(* Logix 5000 Routine export Bead_Edit_Support; software revision 36.00 *)

TYPE DUT_NDSN_spLink :   // UDDT that holds the Cyclic and ACyclic data for the SpectraLink.
STRUCT
   b_r_LostComm : BOOL;
   b_r_PLC_CommReadOnly : BOOL;
   b_r_SystemReady : BOOL;   // Pattern Status Word 0 Bit 0
   b_r_Fault : BOOL;   // Pattern Status Word 0 Bit 1
   b_r_Alert : BOOL;   // Pattern Status Word 0 Bit 2
   b_r_Commissioned : BOOL;   // Pattern Status Word 0 Bit 3
   b_r_RecipeModified : BOOL;   // Pattern Status Word 0 Bit 5
   i_r_Recipe : INT;
   i_r_PalletizedCount : INT;
   i_r_PalletizedSkipCount : INT;
   di_r_App_Trig_ProductCount : DINT;
   di_r_FeedCount : DINT;
   di_r_DeliveryCount : DINT;
   st_r_AppStat : DUT_NDSN_spLink_Chan_Status[8];
   st_r_TrigStat : DUT_NDSN_spLink_Trig_Status[8];
   st_r_EncoStat : DUT_NDSN_spLink_Encoder_Status[8];
   i_r_ProductLength : DINT[8];
   i_r_ProdRate : INT;
   i_r_LineSpeed : INT[2];   // m/min units
   i_r_RunupOutput : INT[2];
   b_w_UnitEnable : BOOL;   // Pattern Control Word 0 Bit 0
   b_w_ClearAllAlarms : BOOL;   // Clear all System Faults and Alerts (Rising Edge).
   b_w_ResetAllCounters : BOOL;   // Reset all counters (rising edge).
   i_w_LoadRecipe : INT;
   i_w_PalletizedCount : INT;   // Write 0 to decrement; 1 to increment; 2 to reset; else does nothing.
   i_w_PalletizedSkipCount : INT;   // Write 0 to decrement; 1 to increment; 2 to reset; else does nothing.
   di_w_App_Trig_ProductCount : DINT;
   di_w_FeedCountReset : DINT;
   di_w_DeliveryCountReset : DINT;
   st_w_AppCtl : DUT_NDSN_spLink_Chan_CTL[8];
   st_rw_BeadAgg : DUT_NDSN_spLink_Bead[8];
   i_rw_RnUpPercentOutP1 : INT[2];
   i_rw_RnUpLineSpdP1 : INT[2];
   i_rw_RnUpPercentOutP2 : INT[2];
   i_rw_RnUpLineSpdP2 : INT[2];
   i_rw_RnUpLowLim : INT[2];
   i_rw_RnUpHighLim : INT[2];
   di_rw_EncoderRes : DINT[2];
   i_rw_TriggerMaskDist : DINT[8];
   i_rw_TriggerChCtl : INT[8];
   i_rw_EncoderChCtl : INT[2];
   i_rw_RandAdjStart : INT[8];
   i_rw_RandAdjEnd : INT[8];
   i_rw_VirtualTriggerSize : DINT[8];
   i_rw_ContStartSpeed : INT[8];
   i_rw_ContStopSpeed : INT[8];
   i_rw_ContKnifeCutDelay : DINT[8];
   i_rw_ContKnifeCutGap : DINT[8];
   di_rw_GTO : DINT[8];
   i_r_ErrorInfo : INT[4];
   i_r_SpecCtl : INT[4];
   i_r_CurrentFault : INT;
END_STRUCT
END_TYPE

TYPE DUT_NDSN_spLink_Bead :
STRUCT
   di_rw_NumOfBeads : DINT;
   di_rw_BeadDelay : DINT[8];   // 1/4 mm
   di_rw_BeadDuration : DINT[8];   // 1/4 mm
   di_rw_mode : DINT;   // 1/4 mm
   di_rw_MaxGunTime : DINT;   // microseconds
   di_rw_LineSpeedActivation : DINT;   // 100th m/min
   di_rw_LineSpeedDeactivation : DINT;   // 100th m/min
   di_rw_Interval : DINT;   // 1/4 mm
   di_rw_AdhesiveSavings : DINT;   // 30%-60%
   di_rw_EcoBeadPattern : DINT;   // 0-40, Illegal values: 0,1,11,20,21,30,31,38,39
END_STRUCT
END_TYPE

TYPE DUT_NDSN_spLink_Chan_CTL :
STRUCT
   b_w_Enable : BOOL;
   b_w_Purge : BOOL;
END_STRUCT
END_TYPE

TYPE DUT_NDSN_spLink_Chan_Status :
STRUCT
   b_r_Enabled : BOOL;
   b_r_Fault : BOOL;
   b_r_Alert : BOOL;
   b_r_Output_Active : BOOL;
   b_r_Installed : BOOL;
END_STRUCT
END_TYPE

TYPE DUT_NDSN_spLink_Encoder_Status :   // SpectraLink Encoder Channel Status
STRUCT
   b_r_Missing : BOOL;
   b_r_Phase_Missing : BOOL;
   b_r_Scaled : BOOL;
   b_r_Fault : BOOL;
   b_r_Alert : BOOL;
   b_r_Installed : BOOL;
END_STRUCT
END_TYPE

TYPE DUT_NDSN_spLink_Trig_Status :   // SpectraLink Trigger Channel Status
STRUCT
   b_r_Detected : BOOL;
   b_r_Fault : BOOL;
   b_r_Alert : BOOL;
   b_r_Active : BOOL;
   b_r_Installed : BOOL;
END_STRUCT
END_TYPE

ADD_ON_INSTRUCTION AOI_Add_Quad_Resolution   (* revision 1.0 *)
// Raw data from the SpectraLink has a x4 factor included for resolution.  This ADI adds that factor for the SpectraLink.
VAR_IN_OUT
   Bead_Agg : DUT_NDSN_spLink_Bead; {required}
END_VAR
VAR_INPUT
   i_Counter : INT; {access Read Only}
END_VAR

ROUTINE Logic   (* structured text *)
// Raw data from the SpectraLink has a x4 factor included for resolution.  This ADI removes that factor to make editing easier.
   //
   //
   
   FOR i_Counter := 0 TO 7 DO
   
   	Bead_Agg.di_rw_BeadDelay[i_Counter] := Bead_Agg.di_rw_BeadDelay[i_Counter]*4;
   	Bead_Agg.di_rw_BeadDuration[i_Counter] := Bead_Agg.di_rw_BeadDuration[i_Counter]*4;
   
   END_FOR;
END_ROUTINE
END_ADD_ON_INSTRUCTION

ADD_ON_INSTRUCTION AOI_Bead_Calculate_Limits   (* revision 1.0 *)
VAR_IN_OUT
   UDDT1 : DUT_NDSN_spLink_Bead; {required}
   di_DelayHi : DINT[8]; {required}
   di_DelayLo : DINT[8]; {required}
   di_DurHi : DINT[8]; {required}
   di_DurLo : DINT[8]; {required}
END_VAR
VAR_INPUT
   b_time_distance_Mode : BOOL; {access Read Only, required}   // Time
END_VAR
VAR_IN_OUT
   i_DotIntervalHi : DINT; {required}
   i_DotIntervalLo : DINT; {required}
END_VAR
VAR
   Max_Hi_Limit : DINT; {access None}
   i_Counter : INT; {access None}
   i_BeadTemp : INT; {access None}
   DotIntHiLimit : INT; {access None}
   DotIntLoLimit : INT; {access None}
END_VAR

ROUTINE Logic   (* structured text *)
   //****************************************************************************************
   //
   //  Subroutine:  Bead_Calculate_Limits
   //
   //  Function:  Calculate the Bead Edit Low and Hi limits for the Delay and Duration.
   //
   //***************************************************************************************
   
   
   //  Init Code
   //
   
   	If (b_time_distance_Mode) Then
   		Max_Hi_Limit := 10000;
   		i_DotIntervalHi := 1000;
   		i_DotIntervalLo := 2;
   	else
   		Max_Hi_Limit := 99999;
   		i_DotIntervalHi := 99999;
   		i_DotIntervalLo := 5;
   	end_if;
   
   	i_BeadTemp := UDDT1.di_rw_NumOfBeads-1;
   
   //
   	FOR i_Counter := 0 TO 7 DO
   
   		If (i_Counter = 0) then			// Special starting Conditions for Lower Delay Limit and High Duration Limit
   			di_DelayLo[i_Counter] := 	0;
   			di_DelayHi[i_Counter] := 	UDDT1.di_rw_BeadDelay[i_Counter + 1] - UDDT1.di_rw_BeadDuration[i_Counter] - 1;
   			di_DurHi[i_Counter] := 		UDDT1.di_rw_BeadDelay[i_Counter + 1] - UDDT1.di_rw_BeadDelay[i_Counter] - 1;
   			di_DurLo[i_Counter] := 		1;			//  ALL Duration Low Limits are set to 1
   		end_if;
   
   		If ((i_Counter < i_BeadTemp) AND (i_Counter > 0)) then
   			di_DelayLo[i_Counter] := 	UDDT1.di_rw_BeadDelay[i_Counter-1] + UDDT1.di_rw_BeadDuration[i_Counter-1] + 1;
   			di_DelayHi[i_Counter] := 	UDDT1.di_rw_BeadDelay[i_Counter + 1] - UDDT1.di_rw_BeadDuration[i_Counter] - 1;
   			di_DurHi[i_Counter] := 		UDDT1.di_rw_BeadDelay[i_Counter + 1] - UDDT1.di_rw_BeadDelay[i_Counter]  - 1;
   			di_DurLo[i_Counter] := 		1;			//  ALL Duration Low Limits are set to 1
   		end_if;
   
   		if ((i_Counter = i_BeadTemp) AND (i_Counter > 0)) then
   			di_DelayLo[i_Counter] := 	UDDT1.di_rw_BeadDelay[i_Counter-1] + UDDT1.di_rw_BeadDuration[i_Counter-1] + 1;
   			di_DelayHi[i_Counter] := 	Max_Hi_Limit;
   			di_DurHi[i_Counter] := 		Max_Hi_Limit;
   			di_DurLo[i_Counter] := 		1;			//  ALL Duration Low Limits are set to 1
   		end_if;
   
   		if ((i_Counter = i_BeadTemp) AND (i_Counter = 0)) then
   			di_DelayLo[i_Counter] := 	0;
   			di_DelayHi[i_Counter] := 	Max_Hi_Limit;
   			di_DurHi[i_Counter] := 		Max_Hi_Limit;
   			di_DurLo[i_Counter] := 		1;			//  ALL Duration Low Limits are set to 1
   		end_if;
   
   		if (i_Counter > i_BeadTemp) then
   			di_DelayLo[i_Counter] := 	0;
   			di_DelayHi[i_Counter] := 	0;
   			di_DurHi[i_Counter] := 		0;
   			di_DurLo[i_Counter] := 		0;
   		end_if;
   
   
   	END_FOR;
END_ROUTINE
END_ADD_ON_INSTRUCTION

ADD_ON_INSTRUCTION AOI_Remove_Quad_Resolution   (* revision 1.0 *)
// Raw data from the SpectraLink has a x4 factor included for resolution.  This ADI removes that factor to make editing easier.
VAR_IN_OUT
   Bead_Agg : DUT_NDSN_spLink_Bead; {required}
END_VAR
VAR_INPUT
   i_Counter : INT; {access Read Only}
END_VAR

ROUTINE Logic   (* structured text *)
// Raw data from the SpectraLink has a x4 factor included for resolution.  This ADI removes that factor to make editing easier.
   //
   //
   
   FOR i_Counter := 0 TO 7 DO
   
   	Bead_Agg.di_rw_BeadDelay[i_Counter] := Bead_Agg.di_rw_BeadDelay[i_Counter]/4;
   	Bead_Agg.di_rw_BeadDuration[i_Counter] := Bead_Agg.di_rw_BeadDuration[i_Counter]/4;
   
   END_FOR;
END_ROUTINE
END_ADD_ON_INSTRUCTION

ADD_ON_INSTRUCTION AOI_UDDT_Compare   (* revision 1.0 *)
VAR_INPUT
   UDDT_INT_SIZE : DINT; {access Read Only, required}
END_VAR
VAR_IN_OUT
   UDDT_1 : DUT_NDSN_spLink_Bead; {required}
   UDDT_2 : DUT_NDSN_spLink_Bead; {required}
END_VAR
VAR_OUTPUT
   NOT_EQUAL : BOOL; {visible}
   EQUAL : BOOL; {visible}
END_VAR
VAR_INPUT
   i_count : INT; {access Read Only}
END_VAR
VAR
   i_buffer1 : DINT[100]; {access None}
   i_buffer2 : DINT[100]; {access None}
   d_count : INT; {access None}
   d_size : INT; {access None}
END_VAR

ROUTINE Logic   (* structured text *)
   //****************************************************************************************************
   //*****  UDDT Compare
   //*****
   //*****  DESCRIPTION:  Subroutine to compare to UDDTs of equal length.  If a difference is located, the NOT_EQUAL output
   //*****					Bit is set.  Otherwise, the EQUAL Bit is set.
   //*****
   //*****
   
   EQUAL := 1;
   NOT_EQUAL := 0;
   i_count := 0;
   d_size := UDDT_INT_SIZE/2;
   
   COP(UDDT_1.di_rw_NumOfBeads, i_buffer1[0], d_size);
   COP(UDDT_2.di_rw_NumOfBeads, i_buffer2[0], d_size);
   
   
   FOR i_count :=0 TO d_size-1 BY 1 DO
   	IF (i_buffer1[i_count] <> i_buffer2[i_count])  THEN
   
   		EQUAL := 0;
   		NOT_EQUAL := 1;
   		EXIT;
   	END_IF;
   END_FOR;
   
END_ROUTINE
END_ADD_ON_INSTRUCTION

VAR_GLOBAL   (* controller tags *)
   b_PView_Edit_PB : BOOL;
   b_PView_EditBeadActive : BOOL;
   b_r_DecrementBeadCh : BOOL;
   b_r_IncrementBeadCh : BOOL;
   b_r_SaveBeadEdits : BOOL;
   Bead_Agg_Temp : DUT_NDSN_spLink_Bead := (di_rw_NumOfBeads := 4, di_rw_BeadDelay[0] := 10, di_rw_BeadDelay[1] := 40, di_rw_BeadDelay[2] := 80, di_rw_BeadDelay[3] := 120, di_rw_BeadDuration[0] := 10, di_rw_BeadDuration[1] := 20, di_rw_BeadDuration[2] := 30, di_rw_BeadDuration[3] := 40, di_rw_mode := 5, di_rw_MaxGunTime := 10000, di_rw_LineSpeedActivation := 500, di_rw_LineSpeedDeactivation := 300, di_rw_Interval := 400, di_rw_AdhesiveSavings := 40, di_rw_EcoBeadPattern := 12);
   BEAD_COMPARE_ADI : AOI_UDDT_Compare := (UDDT_INT_SIZE := 48, EQUAL := 1, i_count := 24);
   di_r_DelayHiLimit : DINT[8] := ([0] := 10000);
   di_r_DelayLowLimit : DINT[8];
   di_r_DurHiLimit : DINT[8] := ([0] := 10000);
   di_r_DurLowLimit : DINT[8] := ([0] := 1);
   i_BeadChannel_Temp : INT;
   i_DotIntervalHi : DINT := 1000;
   i_DotIntervalLo : DINT := 2;
   i_RandomAdjEnd : INT := 40;
   i_RandomAdjEndTemp : INT := 40;
   i_RandomAdjStart : INT := 40;
   i_RandomAdjStartTemp : INT := 40;
   i_rw_BeadChannel : INT;
   ons_decrement : BOOL;
   ons_increment : BOOL;
   spLink_HMI : DUT_NDSN_spLink;
END_VAR

PROGRAM MainProgram
VAR
   ADI_Add_Quad : AOI_Add_Quad_Resolution := (i_Counter := 8);
   ADI_Calc_Limits : AOI_Bead_Calculate_Limits := (b_time_distance_Mode := 1);
   ADI_Remove_Quad : AOI_Remove_Quad_Resolution := (i_Counter := 8);
   ADI_Remove_Quad2 : AOI_Remove_Quad_Resolution := (i_Counter := 8);
   b_EditBeadTemp : BOOL;
   Bead_Agg_Compare : DUT_NDSN_spLink_Bead := (di_rw_NumOfBeads := 4, di_rw_BeadDelay[0] := 10, di_rw_BeadDelay[1] := 40, di_rw_BeadDelay[2] := 80, di_rw_BeadDelay[3] := 120, di_rw_BeadDuration[0] := 10, di_rw_BeadDuration[1] := 20, di_rw_BeadDuration[2] := 30, di_rw_BeadDuration[3] := 40, di_rw_mode := 5, di_rw_MaxGunTime := 10000, di_rw_LineSpeedActivation := 500, di_rw_LineSpeedDeactivation := 300, di_rw_Interval := 400, di_rw_AdhesiveSavings := 40, di_rw_EcoBeadPattern := 12);
   Bead_Agg_Temp2 : DUT_NDSN_spLink_Bead := (di_rw_NumOfBeads := 1, di_rw_BeadDelay[0] := 4, di_rw_BeadDuration[0] := 400, di_rw_mode := 5, di_rw_MaxGunTime := 10000, di_rw_LineSpeedActivation := 500, di_rw_LineSpeedDeactivation := 300, di_rw_Interval := 400, di_rw_AdhesiveSavings := 30, di_rw_EcoBeadPattern := 2);
   Change_Detected : BOOL;
   EditToggle_ONS : BOOL;
END_VAR

ROUTINE Bead_Edit_Support   (* ladder *)
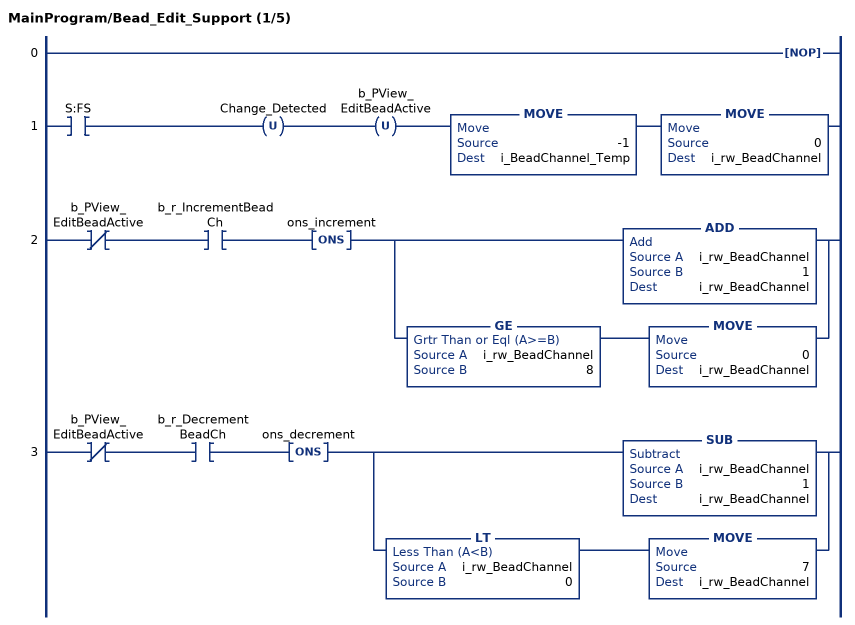
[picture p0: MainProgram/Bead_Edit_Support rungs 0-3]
   0: NOP();
   1: XIC(S:FS)OTU(Change_Detected)OTU(b_PView_EditBeadActive)MOVE(-1,i_BeadChannel_Temp)MOVE(0,i_rw_BeadChannel);
   2: XIO(b_PView_EditBeadActive)XIC(b_r_IncrementBeadCh)ONS(ons_increment)[ADD(i_rw_BeadChannel,1,i_rw_BeadChannel) ,GE(i_rw_BeadChannel,8) MOVE(0,i_rw_BeadChannel) ];
   3: XIO(b_PView_EditBeadActive)XIC(b_r_DecrementBeadCh)ONS(ons_decrement)[SUB(i_rw_BeadChannel,1,i_rw_BeadChannel) ,LT(i_rw_BeadChannel,0) MOVE(7,i_rw_BeadChannel) ];
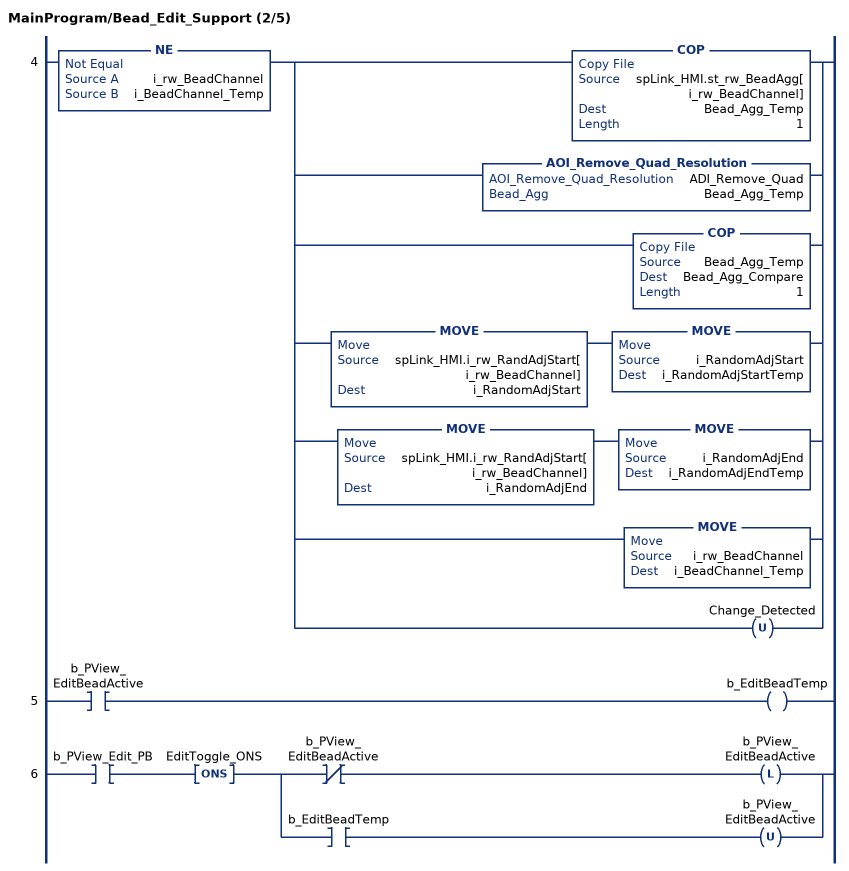
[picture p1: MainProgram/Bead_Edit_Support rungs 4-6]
   4: NE(i_rw_BeadChannel,i_BeadChannel_Temp)[COP(spLink_HMI.st_rw_BeadAgg[ i_rw_BeadChannel],Bead_Agg_Temp,1) ,AOI_Remove_Quad_Resolution(ADI_Remove_Quad,Bead_Agg_Temp) ,COP(Bead_Agg_Temp,Bead_Agg_Compare,1) ,MOVE(spLink_HMI.i_rw_RandAdjStart[i_rw_BeadChannel],i_RandomAdjStart) MOVE(i_RandomAdjStart,i_RandomAdjStartTemp) ,MOVE(spLink_HMI.i_rw_RandAdjStart[i_rw_BeadChannel],i_RandomAdjEnd) MOVE(i_RandomAdjEnd,i_RandomAdjEndTemp) ,MOVE(i_rw_BeadChannel,i_BeadChannel_Temp) ,OTU(Change_Detected) ];
   5: XIC(b_PView_EditBeadActive)OTE(b_EditBeadTemp);
   6: XIC(b_PView_Edit_PB)ONS(EditToggle_ONS)[XIO(b_PView_EditBeadActive) OTL(b_PView_EditBeadActive) ,XIC(b_EditBeadTemp) OTU(b_PView_EditBeadActive) ];
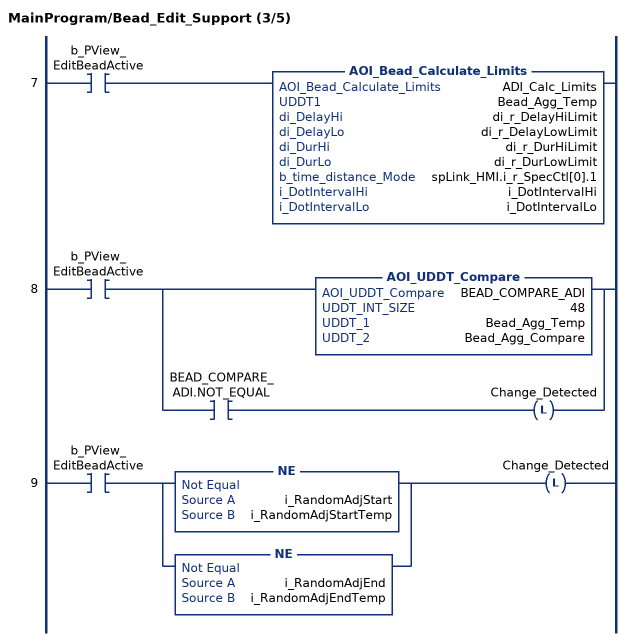
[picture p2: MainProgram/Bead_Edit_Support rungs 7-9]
   7: XIC(b_PView_EditBeadActive)AOI_Bead_Calculate_Limits(ADI_Calc_Limits,Bead_Agg_Temp,di_r_DelayHiLimit,di_r_DelayLowLimit,di_r_DurHiLimit,di_r_DurLowLimit,spLink_HMI.i_r_SpecCtl[0].1,i_DotIntervalHi,i_DotIntervalLo);
   8: XIC(b_PView_EditBeadActive)[AOI_UDDT_Compare(BEAD_COMPARE_ADI,48,Bead_Agg_Temp,Bead_Agg_Compare) ,XIC(BEAD_COMPARE_ADI.NOT_EQUAL) OTL(Change_Detected) ];
   9: XIC(b_PView_EditBeadActive)[NE(i_RandomAdjStart,i_RandomAdjStartTemp) ,NE(i_RandomAdjEnd,i_RandomAdjEndTemp) ]OTL(Change_Detected);
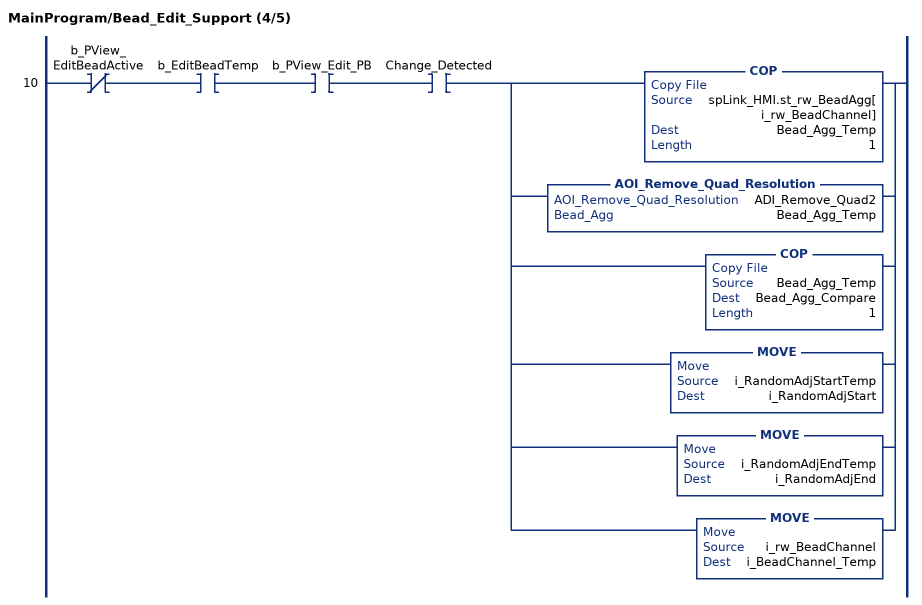
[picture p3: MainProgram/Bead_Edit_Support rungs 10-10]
   10: XIO(b_PView_EditBeadActive)XIC(b_EditBeadTemp)XIC(b_PView_Edit_PB)XIC(Change_Detected)[COP(spLink_HMI.st_rw_BeadAgg[ i_rw_BeadChannel],Bead_Agg_Temp,1) ,AOI_Remove_Quad_Resolution(ADI_Remove_Quad2,Bead_Agg_Temp) ,COP(Bead_Agg_Temp,Bead_Agg_Compare,1) ,MOVE(i_RandomAdjStartTemp,i_RandomAdjStart) ,MOVE(i_RandomAdjEndTemp,i_RandomAdjEnd) ,MOVE(i_rw_BeadChannel,i_BeadChannel_Temp) ];
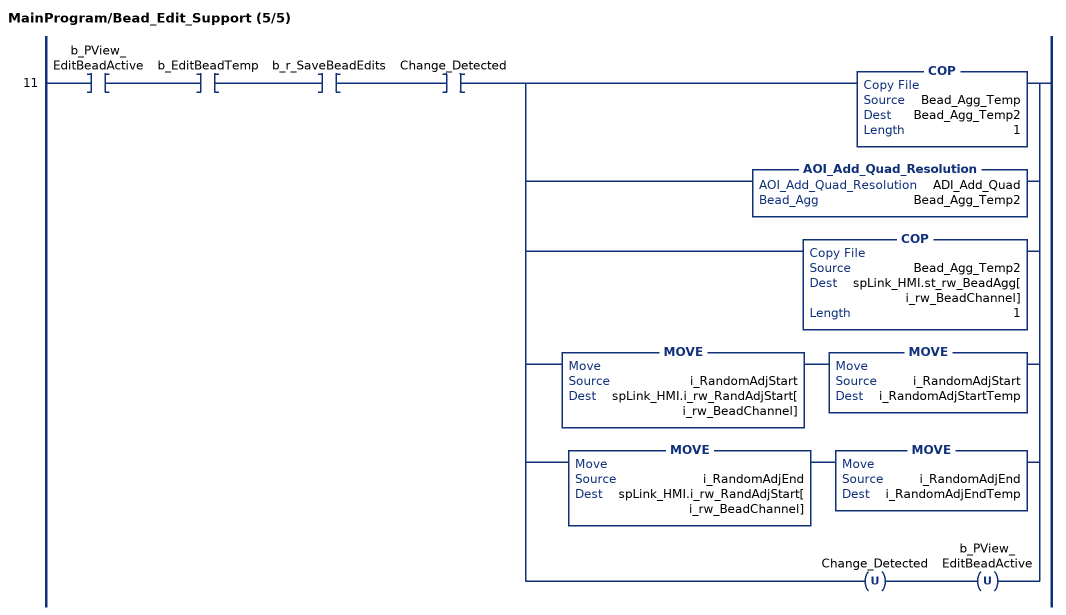
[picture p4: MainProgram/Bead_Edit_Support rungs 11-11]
   11: XIC(b_PView_EditBeadActive)XIC(b_EditBeadTemp)XIC(b_r_SaveBeadEdits)XIC(Change_Detected)[COP(Bead_Agg_Temp,Bead_Agg_Temp2,1) ,AOI_Add_Quad_Resolution(ADI_Add_Quad,Bead_Agg_Temp2) ,COP(Bead_Agg_Temp2,spLink_HMI.st_rw_BeadAgg[ i_rw_BeadChannel],1) ,MOVE(i_RandomAdjStart,spLink_HMI.i_rw_RandAdjStart[i_rw_BeadChannel]) MOVE(i_RandomAdjStart,i_RandomAdjStartTemp) ,MOVE(i_RandomAdjEnd,spLink_HMI.i_rw_RandAdjStart[i_rw_BeadChannel]) MOVE(i_RandomAdjEnd,i_RandomAdjEndTemp) ,OTU(Change_Detected) OTU(b_PView_EditBeadActive) ];
END_ROUTINE
END_PROGRAM
